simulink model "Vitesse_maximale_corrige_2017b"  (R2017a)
settings: Solver=VariableStepAuto  StartTime=0.0  StopTime=20  MinStep=0.00001  RelTol=1e-3
model workspace: external: MAT-File (data not in the file)
libraries: fl_lib x19, nesl_utility x13, sdl_lib x3, powerlib_meascontrol x3, ee_lib x3, batteryecm_lib x1

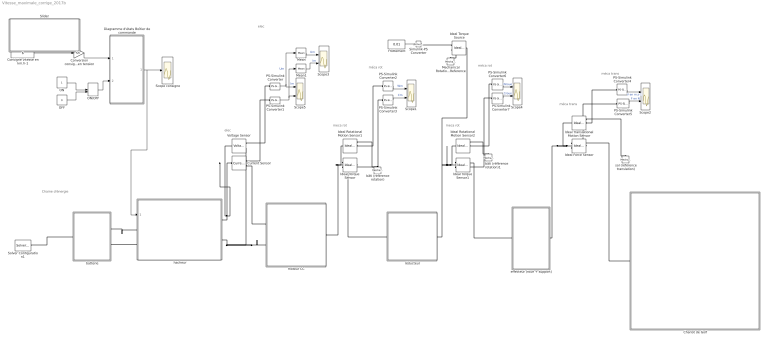
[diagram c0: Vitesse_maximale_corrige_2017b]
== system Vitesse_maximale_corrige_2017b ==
  note: méca rot
  note: méca trans
  note: meca rot
  note: elec
  note: elec
  note: meca rot
  note: Chaine d'énergie
  note: méca trans
  note: méca rot
  Chariot de Golf : Subsystem
  Consigne vitesse en km.h-1 : Constant  Value=6
  Conversion consigne en tension : Gain  Gain=5/6
  Current Sensor : fl_lib/Electrical/Electrical Sensors/Current Sensor
  Diagramme d'états Boîtier de commande : Stateflow chart  TreatAsAtomicUnit=on
  Frottement : Constant  Value=0.01
  Ideal Force Sensor : fl_lib/Mechanical/Mechanical Sensors/Ideal Force Sensor
  Ideal Rotational Motion Sensor1 : fl_lib/Mechanical/Mechanical Sensors/Ideal Rotational Motion Sensor  reference=foundation.enum.MeasurementReference.difference  acceleration_port=false  velocity_port=true  position_port=true  wrap_angle=false  offset=0 rad
  Ideal Rotational Motion Sensor2 : fl_lib/Mechanical/Mechanical Sensors/Ideal Rotational Motion Sensor  reference=foundation.enum.MeasurementReference.difference  acceleration_port=false  velocity_port=true  position_port=true  wrap_angle=false  offset=0 rad
  Ideal Torque Sensor : fl_lib/Mechanical/Mechanical Sensors/Ideal Torque Sensor
  Ideal Torque Sensor1 : fl_lib/Mechanical/Mechanical Sensors/Ideal Torque Sensor
  Ideal Torque Source : fl_lib/Mechanical/Mechanical Sources/Ideal Torque Source
  Ideal Translational Motion Sensor : fl_lib/Mechanical/Mechanical Sensors/Ideal Translational Motion Sensor  reference=foundation.enum.MeasurementReference.difference  acceleration_port=false  velocity_port=true  position_port=true  offset=0 m
  Mean : powerlib_meascontrol/Measurements/Mean  Freq=100  Vinit=24  Ts=0
  Mean1 : powerlib_meascontrol/Measurements/Mean  Freq=100  Vinit=24  Ts=0
  Mechanical Rotational Reference : fl_lib/Mechanical/Rotational Elements/Mechanical Rotational Reference
  OFF : Constant  Value=0
  ON : Constant
  ON/OFF : ManualSwitch
  PS-Simulink Converter : nesl_utility/PS-Simulink Converter  PhysicalDomain=network_engine_domain  SubClassName=ps_output  LeftPortType=input  RightPortType=output  PseudoPeriodic=off  Frequencies=[]  VectorFormat=1-D array  Unit=V  AffineConversion=off
  PS-Simulink Converter1 : nesl_utility/PS-Simulink Converter  PhysicalDomain=network_engine_domain  SubClassName=ps_output  LeftPortType=input  RightPortType=output  PseudoPeriodic=off  Frequencies=[]  VectorFormat=1-D array  Unit=A  AffineConversion=off
  PS-Simulink Converter2 : nesl_utility/PS-Simulink Converter  PhysicalDomain=network_engine_domain  SubClassName=ps_output  LeftPortType=input  RightPortType=output  PseudoPeriodic=off  Frequencies=[]  VectorFormat=1-D array  Unit=rad/s  AffineConversion=off
  PS-Simulink Converter3 : nesl_utility/PS-Simulink Converter  PhysicalDomain=network_engine_domain  SubClassName=ps_output  LeftPortType=input  RightPortType=output  PseudoPeriodic=off  Frequencies=[]  VectorFormat=1-D array  Unit=N*m  AffineConversion=off
  PS-Simulink Converter4 : nesl_utility/PS-Simulink Converter  PhysicalDomain=network_engine_domain  SubClassName=ps_output  LeftPortType=input  RightPortType=output  PseudoPeriodic=off  Frequencies=[]  VectorFormat=1-D array  Unit=m/s  AffineConversion=off
  PS-Simulink Converter5 : nesl_utility/PS-Simulink Converter  PhysicalDomain=network_engine_domain  SubClassName=ps_output  LeftPortType=input  RightPortType=output  PseudoPeriodic=off  Frequencies=[]  VectorFormat=1-D array  Unit=N  AffineConversion=off
  PS-Simulink Converter6 : nesl_utility/PS-Simulink Converter  PhysicalDomain=network_engine_domain  SubClassName=ps_output  LeftPortType=input  RightPortType=output  PseudoPeriodic=off  Frequencies=[]  VectorFormat=1-D array  Unit=rad/s  AffineConversion=off
  PS-Simulink Converter7 : nesl_utility/PS-Simulink Converter  PhysicalDomain=network_engine_domain  SubClassName=ps_output  LeftPortType=input  RightPortType=output  PseudoPeriodic=off  Frequencies=[]  VectorFormat=1-D array  Unit=N*m  AffineConversion=off
  Scope consigne : Scope
  "Scope1 " : Scope  NumInputPorts=2
  "Scope2 " : Scope  NumInputPorts=2
  "Scope3 " : Scope  NumInputPorts=2
  "Scope4 " : Scope  NumInputPorts=2
  "Scope5 " : Scope  NumInputPorts=2
  Simulink-PS Converter : nesl_utility/Simulink-PS Converter  PhysicalDomain=network_engine_domain  SubClassName=ps_input  LeftPortType=input  RightPortType=output  PseudoPeriodic=off  Frequencies=[]  NoiseDistribution=none  NoiseParameters=[]  Unit=N*m  AffineConversion=off  FilteringAndDerivatives=provide  SimscapeFilterOrder=1  InputFilterTimeConstant=0.001  UdotUserProvided=0
  Slider : Subsystem  DialogController=hmiCreateDDGDialog  IsWebBlock=on
  Solver Configuration1 : nesl_utility/Solver Configuration  PhysicalDomain=network_engine_domain  SubClassName=solver  LeftPortType=input  RightPortType=generic  Tones=[]  Harmonics=[]  SimulateNoise=off  Profile=off  UseLocalSampling=off  EnableSwitchedLinearOptims=on  FrequencyDomain=off  UseCCode=off  RelTol=0.001  AbsTol=1e-06  MinStep=1e-09  ToWorkspace=off  RevertToSquareIcSolve=off  NumHomotopyIterations=100  PhasorMode=off  PhasorModeNumHarmonics=1  ConsistencySolver=NEWTON_FTOL  IndexReductionMethod=DerivativeReplacement  DoDC=off  ResidualTolerance=1e-09  ConsistencyTolSource=GLOBAL  ConsistencyAbsTol=0.001  ConsistencyRelTol=0.001  ConsistencyTolFactor=0.001  UseLocalSolver=off  LocalSolverChoice=NE_BACKWARD_EULER_ADVANCER  ResolveIndetEquations=on  FunctionEvalNumThread=1  LocalSolverSampleTime=0.001  DoFixedCost=off  MaxNonlinIter=3  MaxModeIter=2  ComputeImpulses=off  ImpulseIterations=2  LinearAlgebra=Sparse  LinearAlgebraNumThread=0  EquationFormulation=NE_TIME_EF  DelaysMemoryBudget=1024  AutomaticFiltering=on  FilteringTimeConstant=0.001  PartitionStorageMethod=AS_NEEDED  PartitionMemoryBudget=1024  PartitionMethod=FAST  MultibodyUseLocalSolver=off  MultibodyLocalSolverChoice=ODE1  MultibodyLocalSolverSampleTime=0.001
  Voltage Sensor : fl_lib/Electrical/Electrical Sensors/Voltage Sensor
  batterie : Subsystem
  bâti (référence rotation) : fl_lib/Mechanical/Rotational Elements/Mechanical Rotational Reference
  bâti (référence rotation)1 : fl_lib/Mechanical/Rotational Elements/Mechanical Rotational Reference
  effecteur (roue + support) : Subsystem
  hacheur : Subsystem
  moteur CC : Subsystem
  réducteur : Subsystem
  sol (référence translation) : fl_lib/Mechanical/Translational Elements/Mechanical Translational Reference
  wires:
  PS-Simulink Converter1/1 -> Mean1/1, "Scope5 "/2  "Im"
  PS-Simulink Converter4/1 -> "Scope2 "/1  "V en m.s-1"
  Mean/1 -> "Scope3 "/1  "Um"
  PS-Simulink Converter/1 -> Mean/1, "Scope5 "/1  "Um"
  Mean1/1 -> "Scope3 "/2  "Im"
  PS-Simulink Converter5/1 -> "Scope2 "/2  "F en N"
  PS-Simulink Converter2/1 -> "Scope1 "/1  "Wm"
  PS-Simulink Converter6/1 -> "Scope4 "/1  "Wroue"
  PS-Simulink Converter3/1 -> "Scope1 "/2  "Cm"
  Frottement/1 -> Simulink-PS Converter/1
  PS-Simulink Converter7/1 -> "Scope4 "/2  "Croue"
  Diagramme d'états Boîtier de commande/1(consigne) -> hacheur/1(Consigne), Scope consigne/1
  ON/1 -> ON/OFF/1
  ON/OFF/1 -> Diagramme d'états Boîtier de commande/2(Bouton_marche)
  OFF/1 -> ON/OFF/2
  Conversion consigne en tension/1 -> Diagramme d'états Boîtier de commande/1(Potentiometre)
  Consigne vitesse en km.h-1/1 -> Conversion consigne en tension/1
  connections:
  hacheur/RConn2 -- moteur CC/LConn2 -- Voltage Sensor/RConn2
  Ideal Force Sensor/LConn1 -- Ideal Translational Motion Sensor/LConn1 -- effecteur (roue + support)/RConn1
  hacheur/RConn1 -- Current Sensor/LConn1 -- Voltage Sensor/LConn1
  Ideal Torque Sensor1/LConn1 -- Ideal Torque Source/LConn1 -- Ideal Rotational Motion Sensor2/LConn1 -- réducteur/RConn1
  Ideal Torque Sensor/LConn1 -- Ideal Rotational Motion Sensor1/LConn1 -- moteur CC/RConn1
  Ideal Torque Source/RConn2 -- Mechanical Rotational Reference/LConn1
  Ideal Torque Sensor1/RConn1 -- effecteur (roue + support)/LConn1
  Simulink-PS Converter/RConn1 -- Ideal Torque Source/RConn1
  Solver Configuration1/RConn1 -- batterie/LConn1
  Ideal Force Sensor/RConn2 -- PS-Simulink Converter5/LConn1
  batterie/RConn1 -- hacheur/LConn1
  Ideal Rotational Motion Sensor2/RConn1 -- bâti (référence rotation)1/LConn1
  PS-Simulink Converter7/LConn1 -- Ideal Torque Sensor1/RConn2
  Ideal Translational Motion Sensor/RConn2 -- PS-Simulink Converter4/LConn1
  Ideal Translational Motion Sensor/RConn1 -- sol (référence translation)/LConn1
  PS-Simulink Converter6/LConn1 -- Ideal Rotational Motion Sensor2/RConn2
  Current Sensor/RConn2 -- moteur CC/LConn1
  PS-Simulink Converter3/LConn1 -- Ideal Torque Sensor/RConn2
  PS-Simulink Converter2/LConn1 -- Ideal Rotational Motion Sensor1/RConn2
  Ideal Torque Sensor/RConn1 -- réducteur/LConn1
  Ideal Rotational Motion Sensor1/RConn1 -- bâti (référence rotation)/LConn1
  hacheur/LConn2 -- batterie/RConn2
  PS-Simulink Converter1/LConn1 -- Current Sensor/RConn1
  PS-Simulink Converter/LConn1 -- Voltage Sensor/RConn1
  Chariot de Golf/LConn1 -- Ideal Force Sensor/RConn1

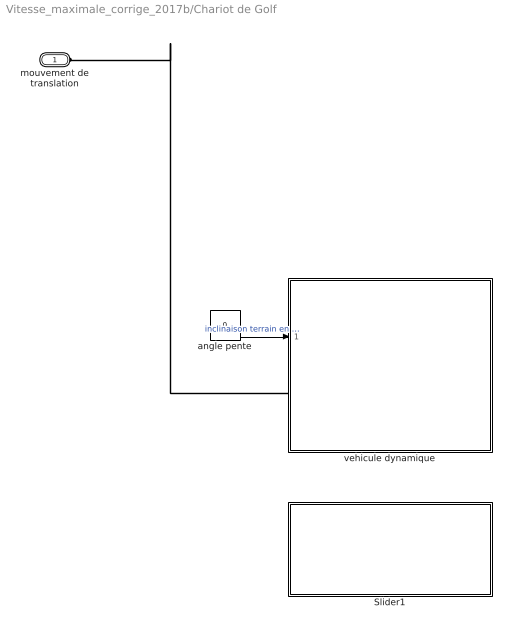
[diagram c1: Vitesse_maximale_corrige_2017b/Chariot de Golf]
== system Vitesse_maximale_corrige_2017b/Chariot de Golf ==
  Slider1 : Subsystem  DialogController=hmiCreateDDGDialog  IsWebBlock=on
  angle pente : Constant  Value=0
  vehicule dynamique : Subsystem
  mouvement de translation : PMIOPort  Side=Left
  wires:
  angle pente/1 -> vehicule dynamique/1(angle pente)  "inclinaison terrain en deg"
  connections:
  vehicule dynamique/LConn1 -- mouvement de translation/RConn1

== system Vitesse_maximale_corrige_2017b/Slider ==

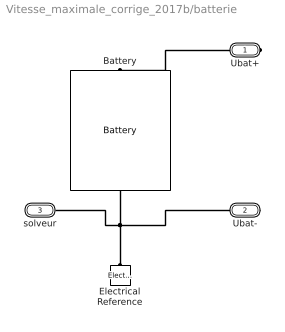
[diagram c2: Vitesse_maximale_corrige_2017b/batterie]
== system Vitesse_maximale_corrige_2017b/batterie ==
  Battery : batteryecm_lib/Battery  Vnom=16.5 V  prm_dir=simscape.enum.battery.prm_dir.disabled  R1_dis=2 Ohm  R1_ch=2 Ohm  R1=0.1 Ohm  prm_AH=2  AH=16 hr*A  V1=11.84 V  AH1=12.8 hr*A  prm_R2=2  R2=inf Ohm  Tmeas=298.15 K  charge_measurement_port=simscape.enum.battery.enable.no  prm_dyn=1  Rp1=0.005 Ohm  tau1=30 s  Rp2=0.005 Ohm  tau2=30 s  Rp3=0.005 Ohm  tau3=30 s  Rp4=0.005 Ohm  tau4=30 s  Rp5=0.005 Ohm  tau5=30 s  prm_fade=1  N_fade=100  AH_fade=45 hr*A  R1_fade=2.02 Ohm  R1_ch_fade=2.02 Ohm  V1_fade=10.35 V  prm_age=simscape.enum.battery.prm_age.disabled  prm_age_OCV=simscape.enum.battery.prm_age_OCV.OCV  OCV_age=0.9  SOC_age=60  Tmeas_age=298.15 K  delta_time_age_vec=[0] d  temperature_age_vec=[273] K  OCV_scaling_age=2.2134e6  OCV_offset_age=1.632e6  temp_exp_age=0.515833569 V  t_exp_age=0.75  Vnom_T2=12 V  R1_T2=2.2 Ohm  R1_T2_dis=2.2 Ohm  R1_T2_ch=2.2 Ohm  V1_T2=11.4 V  R2_T2=2200 Ohm  Rp1_T2=0.005 Ohm  tau1_T2=30 s  Rp2_T2=0.005 Ohm  tau2_T2=30 s  Rp3_T2=0.005 Ohm  tau3_T2=30 s  Rp4_T2=0.005 Ohm  tau4_T2=30 s  Rp5_T2=0.005 Ohm  tau5_T2=30 s  Tmeas2=273.15 K  thermal_port=simscape.enum.thermaleffects.omit  thermal_mass=30000 J/K  i_specify=off  i_priority=None  i=0 A  i_nominal_specify=off  i_nominal_unit=A  i_nominal_value=1  v_specify=off  v_priority=None  v=0 V  v_nominal_specify=off  v_nominal_unit=V  v_nominal_value=1  charge_specify=on  charge_priority=High  charge=17 hr*A  charge_nominal_specify=off  charge_nominal_unit=A*hr  charge_nominal_value=1  num_cycles_specify=on  num_cycles_priority=High  num_cycles=1  num_cycles_nominal_specify=off  num_cycles_nominal_unit=1  num_cycles_nominal_value=1  temperature_specify=off  temperature_priority=High  temperature=298.15 K  temperature_nominal_specify=off  temperature_nominal_unit=K  temperature_nominal_value=1
  Electrical Reference : fl_lib/Electrical/Electrical Elements/Electrical Reference
  Ubat+ : PMIOPort  Side=Right
  Ubat- : PMIOPort  Port=2  Side=Right
  solveur : PMIOPort  Port=3  Side=Left
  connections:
  Electrical Reference/LConn1 -- solveur/RConn1 -- Ubat-/RConn1 -- Battery/RConn1
  Ubat+/RConn1 -- Battery/LConn1

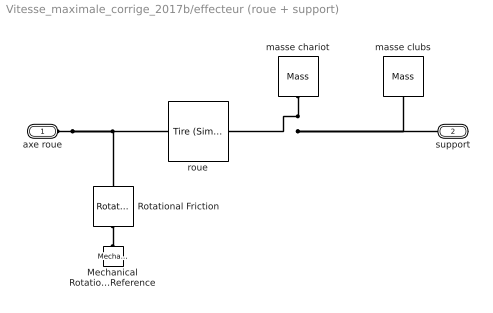
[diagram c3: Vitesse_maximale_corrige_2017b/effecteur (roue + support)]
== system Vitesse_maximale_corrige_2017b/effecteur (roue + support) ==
  Mechanical Rotational Reference : fl_lib/Mechanical/Rotational Elements/Mechanical Rotational Reference
  "Rotational Friction " : fl_lib/Mechanical/Rotational Elements/Rotational Friction  brkwy_trq=0.1 N*m  brkwy_vel=0.1 rad/s  Col_trq=0.1 N*m  visc_coef=0.0001 N*m/(rad/s)  w_specify=off  w_priority=None  w=0 rad/s  w_nominal_specify=off  w_nominal_unit=rad/s  w_nominal_value=1  t_specify=off  t_priority=None  t=0 N*m  t_nominal_specify=off  t_nominal_unit=N*m  t_nominal_value=1
  masse clubs : fl_lib/Mechanical/Translational Elements/Mass  mass=4 kg  num_ports=foundation.enum.numPorts2.one  v_specify=off  v_priority=High  v=0 m/s  v_nominal_specify=off  v_nominal_unit=m/s  v_nominal_value=1  f_specify=off  f_priority=High  f=0 N  f_nominal_specify=off  f_nominal_unit=N  f_nominal_value=1
  masse chariot : fl_lib/Mechanical/Translational Elements/Mass  mass=13.5 kg  num_ports=foundation.enum.numPorts2.one  v_specify=off  v_priority=High  v=0 m/s  v_nominal_specify=off  v_nominal_unit=m/s  v_nominal_value=1  f_specify=off  f_priority=High  f=0 N  f_nominal_specify=off  f_nominal_unit=N  f_nominal_value=1
  roue : sdl_lib/Tires & Vehicles/Tire (Simple)  r_tire=27/2 cm  model_compliance=0  stiffness=1e+6 N/m  damping=1000 N/(m/s)  model_inertia=0  tire_inertia=1 kg*m^2  initial_velocity=0 rad/s
  axe roue : PMIOPort  Side=Left
  support : PMIOPort  Port=2  Side=Right
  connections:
  masse chariot/LConn1 -- support/RConn1 -- masse clubs/LConn1 -- roue/RConn1
  axe roue/RConn1 -- roue/LConn1 -- "Rotational Friction "/LConn1
  "Rotational Friction "/RConn1 -- Mechanical Rotational Reference/LConn1

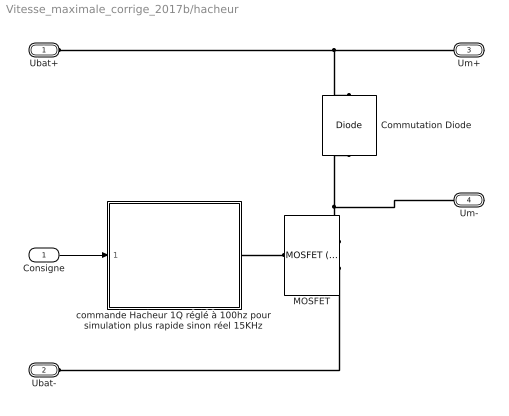
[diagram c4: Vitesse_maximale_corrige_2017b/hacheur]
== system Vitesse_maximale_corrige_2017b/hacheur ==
  Consigne : Inport
  Commutation Diode : ee_lib/Semiconductors & Converters/Diode  ModelType=ee.enum.diode.modelType.pwl  TableType=ee.enum.diode.tableType.IfMat  IfMat=[.07, .12, .19, 1.75, 4.24, 7.32, 11.2; .16, .3, .72, 2.14, 5.02, 8.35, 13.12] A  VfMat=[.9, 1.15, 1.25, 1.5, 1.75, 2.17, 2.6, 2.85; .58, .68, .75, 1.1, 1.38, 1.77, 2.27, 2.7] V  TjVec=[25, 125] degC  VfVec=[.5, .7, .9, 1.3, 1.7, 2.1, 2.5] V  IfVec=[.1, .2, .5, 1, 2, 4, 7, 10] A  Vf=0.8 V  Ron=0.001 Ohm  Goff=1e-5 1/Ohm  prmExp=ee.enum.diode.expParam.useTwo  I12=[.0137, .545] A  V12=[.6, .7] V  RS=0 Ohm  Tmeas=25 degC  IS=1e-12 A  ec=1  I1=0.0137 A  V1=0.6 V  N_series=1  N_parallel=1  ZenerEnable=false  Rz=0.3 Ohm  BV=inf V  C_param=ee.enum.diode.capParam.fixed  CJ=50 pF  CJ0=5 pF  Vvec=[.1, 10, 100] V  Cvec=[3.5, 1, .4] pF  VJ=1 V  Mgrad=0.5  FC=0.5  Q_param=1  iRM=-235 A  iF=300 A  didt=-50 A/us  trr_factor=3  trr=15 us  Qrr=1.5e+3 s*uA  Vr=-600 V  Ls=150 nH  Erec=0.03 J  TT=50 ns  tau=100 ns  T_param=ee.enum.diode.temperatureParam.off  Tdevice=25 degC  I1_T2=0.245 A  V1_T2=0.5 V  IS_T2=1.25e-7 A  Tmeas2=125 degC  XTI_param=ee.enum.diode.xtiParam.pn  XTI=3  EG_param=ee.enum.diode.egapParam.material_si  EG=1.11 eV  dBVdT=0 V/K  enable_faults=ee.enum.enable.no  fault_action=simscape.enum.assert.action.none  fault_types=ee.enum.diode.faults.open  tau_fault=1e-3 s  IfMat_faulted=[.07, .12, .19, 1.75, 4.24, 7.32, 11.2; .16, .3, .72, 2.14, 4.02, 6.35, 9.12] A  VfMat_faulted=[.9, 1.15, 1.25, 1.5, 1.75, 2.17, 2.6, 2.85; .58, .68, .75, 1.1, 1.38, 1.77, 2.27, 2.7] V  VfVec_faulted=[.5, .7, .9, 1.3, 1.7, 2.1, 2.5] V  IfVec_faulted=[.1, .2, .5, 1, 2, 4, 7, 10] A  Ropen_faulted=1000 Ohm  Gshort_faulted=1000 1/Ohm  Vf_faulted=0.6 V  Ron_faulted=0.3 Ohm  Goff_faulted=1e-8 S  I12_faulted=[.0137, .545] A  V12_faulted=[.6, .7] V  IS_faulted=1e-12 A  ec_faulted=1  I1_faulted=0.0137 A  V1_faulted=0.6 V  RS_faulted=0 Ohm  Rz_faulted=0.3 Ohm  BV_faulted=inf V  Cscale_faulted=100  fault_trigger=ee.enum.faults.faultTrigger.temporal  t_fault=inf s  max_permissible_voltage=inf V  n_fail_on_voltage=1  max_permissible_current=inf A  t_fail_on_current=1 s  max_permissible_dVdt=inf V/s  enable_fault_input=simscape.enum.onoff.off  i_specify=off  i_priority=None  i=0 A  i_nominal_specify=off  i_nominal_unit=A  i_nominal_value=1  v_specify=off  v_priority=None  v=0 V  v_nominal_specify=off  v_nominal_unit=V  v_nominal_value=1  v_capacitor_specify=off  v_capacitor_priority=None  v_capacitor=0 V  v_capacitor_nominal_specify=off  v_capacitor_nominal_unit=V  v_capacitor_nominal_value=1  faulted_specify=off  faulted_priority=None  faulted=0  faulted_nominal_specify=off  faulted_nominal_unit=1  faulted_nominal_value=1  i_diode_specify=off  i_diode_priority=None  i_diode=0 A  i_diode_nominal_specify=off  i_diode_nominal_unit=A  i_diode_nominal_value=1  v_diode_specify=off  v_diode_priority=None  v_diode=0 V  v_diode_nominal_specify=off  v_diode_nominal_unit=V  v_diode_nominal_value=1  i_capacitor_specify=off  i_capacitor_priority=None  i_capacitor=0 A  i_capacitor_nominal_specify=off  i_capacitor_nominal_unit=A  i_capacitor_nominal_value=1  power_dissipated_specify=off  power_dissipated_priority=None  power_dissipated=0 W  power_dissipated_nominal_specify=off  power_dissipated_nominal_unit=W  power_dissipated_nominal_value=1  fidelity_level=ee.enum.diode.fidelity.includeChargeDyn  rec_loss_model=ee.enum.diode.reverseRecoveryModel.fixed  ErecVal=0 J  scaleWithIandV=true  ErecMat=zeros(2, 3) J  TjrecVec=[298.15, 398.15] K  IfrecVec=[.1, 1, 10] A  IrecVal=10 A  VrecVal=10 V  tFilter=1 / 1000 / 100 s  max_permissible_temperature=inf K  t_fail_on_temperature=1 s  thermal_network_parameterization=ee.enum.thermalNetworkTopology.junctionCase  Rth=[0, 10] K/W  Rth_Cauer=[1, 3, 10] K/W  Rth_Foster=[4, 6] K/W  thermal_mass_parameterization=ee.enum.thermalNetwork.timeconstant  thermal_mass=[0, 1] J/K  thermal_mass_Cauer=[.1, .3, 1] J/K  thermal_mass_Foster=[1.5, 3] J/K  thermal_time_constant=[0, 10] s  thermal_time_constant_Cauer=[1, 3, 10] s  thermal_time_constant_Foster=[6, 18] s  thermal_mass_initial_temperatures=[25, 25] degC  thermal_mass_initial_temperatures_Cauer=[25, 25, 25] degC  junction_thermal_mass=0.01 J/K  Tvec_initial_Foster=[25, 25, 25, 25] degC  no_thermal_network=0  junction_temperature_specify=off  junction_temperature_priority=None  junction_temperature=25 degC  junction_temperature_nominal_specify=off  junction_temperature_nominal_unit=degC  junction_temperature_nominal_value=1
  MOSFET : ee_lib/Semiconductors & Converters/MOSFET (Ideal, Switching)  port_option=ee.enum.controlport.ps  Rds=0.01 Ohm  Goff=1e-6 1/Ohm  Vth=2 V  diode_param=2  diode_Vf=0.8 V  diode_Ron=0.001 Ohm  diode_Goff=1e-5 1/Ohm  diode_C=5e-8 F  diode_iRM=-235 A  diode_iF=300 A  diode_idot=-50 A/us  diode_trr_param=1  diode_trr_factor=3  diode_trr=15 us  diode_Qrr=1.5e+3 s*uA  ids_specify=off  ids_priority=None  ids=0 A  ids_nominal_specify=off  ids_nominal_unit=A  ids_nominal_value=1  vds_specify=off  vds_priority=None  vds=0 V  vds_nominal_specify=off  vds_nominal_unit=V  vds_nominal_value=1  vgs_specify=off  vgs_priority=None  vgs=0 V  vgs_nominal_specify=off  vgs_nominal_unit=V  vgs_nominal_value=1  thermal_loss_option=ee.enum.converters.thermalLossOption.constantvalues  Von_data=[0, 1.8, 3.2, 6, 10, 16; 0, 2, 5.5, 9.5, 15, 25] V  Tj=[298.15, 448.15] K  Iout_data=[0, 20, 40, 60, 80, 100] A  Eon_data=[0, 55.04, 124.57, 235.53, 362.12; 0, 71.25, 161.25, 304.88, 468.75] * 1e-6 J  Eoff_data=[0, 18, 30, 56.1, 76.5; 0, 22.5, 37.5, 70.13, 95.63] * 1e-6 J  Eon_data_3D=[zeros(2, 5, 3)] J  Eoff_data_3D=[zeros(2, 5, 3)] J  Tj_loss=[298.15, 448.15] K  Iout_data_loss=[0, 10, 20, 30, 40] A  tabulateWithVds=false  Vds_loss=[0, 150, 300] V  Eon_scalar=22.86e-3 J  Eoff_scalar=17.14e-3 J  Voff=300 V  Iout_scalar=600 A  useCurrentFromPreviousCycle=false  useVoltageFromPreviousCycle=false  diodeModelType=ee.enum.converters.diodeModelType.pwl  diodeTableType=ee.enum.diode.tableType.IfMat  diode_IfMat=[.07, .12, .19, 1.75, 4.24, 7.32, 11.2; .16, .3, .72, 2.14, 4.02, 6.35, 9.12] A  diode_VfMat=[.9, 1.15, 1.25, 1.5, 1.75, 2.17, 2.6, 2.85; .58, .68, .75, 1.1, 1.38, 1.77, 2.27, 2.7] V  diode_TjVec=[25, 125] degC  diode_VfVec=[.5, .7, .9, 1.3, 1.7, 2.1, 2.5] V  diode_IfVec=[.1, .2, .5, 1, 2, 4, 7, 10] A  diode_Vr=-600 V  diode_Ls=150 nH  diode_Erec=0.03 J  diode_rec_loss_model=ee.enum.diode.reverseRecoveryModel.fixed  diode_ErecVal=0 J  diode_scaleWithIandV=true  diode_ErecMat=zeros(2, 3) J  diode_TjrecVec=[298.15, 398.15] K  diode_IfrecVec=[.1, 1, 10] A  diode_IrecVal=10 A  diode_VrecVal=10 V  diode_tFilter=1 / 1000 / 100 s  thermal_network_parameterization=ee.enum.thermalNetworkTopology.external  Rth=[.03, .2] K/W  Rth_Cauer=[.03, .1, .2] K/W  Rth_Foster=[.03, .2] K/W  thermal_mass_parameterization=ee.enum.thermalNetwork.timeconstant  thermal_mass=[3, 25] J/K  thermal_mass_Cauer=[3, 10, 25] J/K  thermal_mass_Foster=[33, 50] J/K  thermal_time_constant=[.1, 5] s  thermal_time_constant_Cauer=[.1, 1, 5] s  thermal_time_constant_Foster=[1, 10] s  thermal_mass_initial_temperatures=[25, 25] degC  thermal_mass_initial_temperatures_Cauer=[25, 25, 25] degC  junction_thermal_mass=0.1 J/K  Tvec_initial_Foster=[25, 25, 25, 25] degC  no_thermal_network=0  junction_temperature_specify=off  junction_temperature_priority=None  junction_temperature=25 degC  junction_temperature_nominal_specify=off  junction_temperature_nominal_unit=degC  junction_temperature_nominal_value=1  Qj_specify=off  Qj_priority=None  Qj=0 W  Qj_nominal_specify=off  Qj_nominal_unit=W  Qj_nominal_value=1  accumulatedSwitchingLosses_specify=off  accumulatedSwitchingLosses_priority=None  accumulatedSwitchingLosses=0 J
  commande Hacheur 1Q réglé à 100hz pour simulation plus rapide sinon réel 15KHz : Subsystem
  Ubat+ : PMIOPort  Side=Left
  Ubat- : PMIOPort  Port=2  Side=Left
  Um+ : PMIOPort  Port=3  Side=Right
  Um- : PMIOPort  Port=4  Side=Right
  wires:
  Consigne/1 -> commande Hacheur 1Q réglé à 100hz pour simulation plus rapide sinon réel 15KHz/1(consigne)
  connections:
  Ubat+/RConn1 -- Um+/RConn1 -- Commutation Diode/RConn1
  MOSFET/RConn1 -- Commutation Diode/LConn1 -- Um-/RConn1
  MOSFET/LConn1 -- commande Hacheur 1Q réglé à 100hz pour simulation plus rapide sinon réel 15KHz/RConn1
  MOSFET/RConn2 -- Ubat-/RConn1

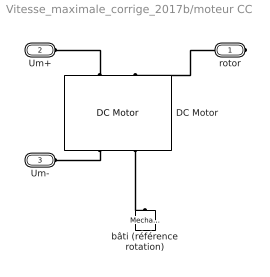
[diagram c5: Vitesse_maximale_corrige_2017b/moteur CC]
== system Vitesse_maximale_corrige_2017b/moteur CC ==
  DC Motor : ee_lib/Electromechanical/Brushed Motors/DC Motor  field_option=ee.enum.field_option.pm  Rf=100 Ohm  Lf=1 H  Laf=0.15 H  If0=0 A  parameterization=1  Ra=0.54 Ohm  La=12e-3 H  emf_or_torque=1  Kv=2.9e-3 V/rpm  Ki=6.876e-4 N*m/A  T_stall=2.4e-4 N*m  w_max=3800 rpm  w_rated=3800 rpm  P_rated=150 W  V_rated=12 V  lam_param=1  i_noload=1 A  V_i_noload=12 V  J=0.0001 kg*m^2  lam=0.0001 N*m/(rad/s)  speed0=0 rpm  enable_fault_armature=simscape.enum.onoff.off  rev_faulted=1 / 3  G_faulted_armature=1e-5 S  fault_trigger_armature=ee.enum.faults.faultTrigger.temporal  t_fault_armature=1 s  max_permissible_current_armature=inf A  t_fail_on_current_armature=1 s  enable_fault_field=simscape.enum.onoff.off  G_faulted_field=1e-5 S  fault_trigger_field=ee.enum.faults.faultTrigger.temporal  t_fault_field=1 s  max_permissible_current_field=inf A  t_fail_on_current_field=1 s  fault_action=simscape.enum.assert.action.none  alpha=3.93e-3 1/K  Tmeas=25 degC  thermal_mass=100 J/K  initial_temperature=25 degC
  bâti (référence rotation) : fl_lib/Mechanical/Rotational Elements/Mechanical Rotational Reference
  rotor : PMIOPort  Side=Right
  Um+ : PMIOPort  Port=2  Side=Left
  Um- : PMIOPort  Port=3  Side=Left
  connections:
  rotor/RConn1 -- DC Motor/LConn2
  DC Motor/RConn2 -- bâti (référence rotation)/LConn1
  DC Motor/RConn1 -- Um-/RConn1
  DC Motor/LConn1 -- Um+/RConn1

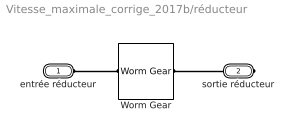
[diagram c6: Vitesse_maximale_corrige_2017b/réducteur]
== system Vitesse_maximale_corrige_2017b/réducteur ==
  Worm Gear : sdl_lib/Gears/Worm Gear  ratio=25/1  thread_type=1  friction_model=2  friction_parameterization=1  pr_ang=20 deg  lead_ang=74.534 deg  fr_coeff=0.08  eff_wg=0.74  eff_gw=0.65  temperature_TLU=[280, 300, 320] K  efficiency_wg_TLU=[.75, .65, .6]  efficiency_gw_TLU=[.5, .45, .4]  pwr_thr=0.001 W  mu_visc=[0, 0] N*m/(rad/s)  thermal_mass=50 J/K  temperature_specify=off  temperature_priority=High  temperature=300 K  temperature_nominal_specify=off  temperature_nominal_unit=K  temperature_nominal_value=1
  entrée réducteur : PMIOPort  Side=Left
  sortie réducteur : PMIOPort  Port=2  Side=Right
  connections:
  entrée réducteur/RConn1 -- Worm Gear/LConn1
  Worm Gear/RConn1 -- sortie réducteur/RConn1

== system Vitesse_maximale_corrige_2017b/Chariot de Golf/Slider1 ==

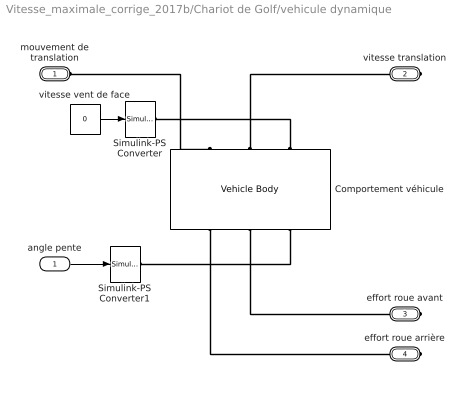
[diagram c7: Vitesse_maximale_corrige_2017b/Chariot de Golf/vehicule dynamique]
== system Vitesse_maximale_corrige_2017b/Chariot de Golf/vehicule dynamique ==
  angle pente : Inport  OutMin=[0]  OutMax=[20000]
  Comportement véhicule : sdl_lib/Tires & Vehicles/Vehicle Body  mass=17.5 kg  n_w=1  x_f=580 mm  x_r=60 mm  y_c=24+27/2 cm  mass_var=simscape.enum.onoff.off  g=9.81 m/s^2  liftoff_warning=0  area=0.52828 m^2  Cd=1  rho=1.24 kg/m^3  model_pitch=0  inertia=4000 kg*m^2  suspension_model=1  k_f=1e4 N/m  b_f=1e4 N/(m/s)  k_r=1e4 N/m  b_r=1e4 N/(m/s)  k_f_TLU=[-2000, -1000, 0, 1000, 2000] N  x_f_TLU=[-.4, -.2, 0, .2, .4] m  b_f_TLU=[-200, -100, 0, 100, 200] N  v_f_TLU=[-4, -2, 0, 2, 4] m/s  k_r_TLU=[-2000, -1000, 0, 1000, 2000] N  x_r_TLU=[-.4, -.2, 0, .2, .4] m  b_r_TLU=[-200, -100, 0, 100, 200] N  v_r_TLU=[-4, -2, 0, 2, 4] m/s  interp_method=simscape.enum.interpolation.linear  extrap_method=simscape.enum.extrapolation.linear  model_hardstop=0  upper_bound_f=.25 m  lower_bound_f=-.25 m  stop_k_f=1e6 N/m  stop_b_f=150 N/(m/s)  upper_bound_r=.25 m  lower_bound_r=-.25 m  stop_k_r=1e6 N/m  stop_b_r=150 N/(m/s)  initial_pitch=0 rad  initial_pitch_rate=0 rad/s  v_specify=on  v_priority=High  v=0 m/s  v_nominal_specify=off  v_nominal_unit=m/s  v_nominal_value=1
  Simulink-PS Converter : nesl_utility/Simulink-PS Converter  PhysicalDomain=network_engine_domain  SubClassName=ps_input  LeftPortType=input  RightPortType=output  PseudoPeriodic=off  Frequencies=[]  NoiseDistribution=none  NoiseParameters=[]  Unit=m/s  AffineConversion=off  FilteringAndDerivatives=zero  SimscapeFilterOrder=1  InputFilterTimeConstant=0.001  UdotUserProvided=1
  Simulink-PS Converter1 : nesl_utility/Simulink-PS Converter  PhysicalDomain=network_engine_domain  SubClassName=ps_input  LeftPortType=input  RightPortType=output  PseudoPeriodic=off  Frequencies=[]  NoiseDistribution=none  NoiseParameters=[]  Unit=deg  AffineConversion=off  FilteringAndDerivatives=zero  SimscapeFilterOrder=1  InputFilterTimeConstant=0.001  UdotUserProvided=1
  vitesse vent de face : Constant  Value=0
  mouvement de translation : PMIOPort  Side=Left
  vitesse translation : PMIOPort  Port=2  Side=Right
  effort roue avant : PMIOPort  Port=3  Side=Right
  effort roue arrière : PMIOPort  Port=4  Side=Right
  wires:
  vitesse vent de face/1 -> Simulink-PS Converter/1
  angle pente/1 -> Simulink-PS Converter1/1
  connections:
  mouvement de translation/RConn1 -- Comportement véhicule/LConn1
  Simulink-PS Converter/RConn1 -- Comportement véhicule/LConn3
  Comportement véhicule/LConn2 -- vitesse translation/RConn1
  Comportement véhicule/RConn2 -- effort roue avant/RConn1
  Comportement véhicule/RConn1 -- effort roue arrière/RConn1
  Simulink-PS Converter1/RConn1 -- Comportement véhicule/RConn3

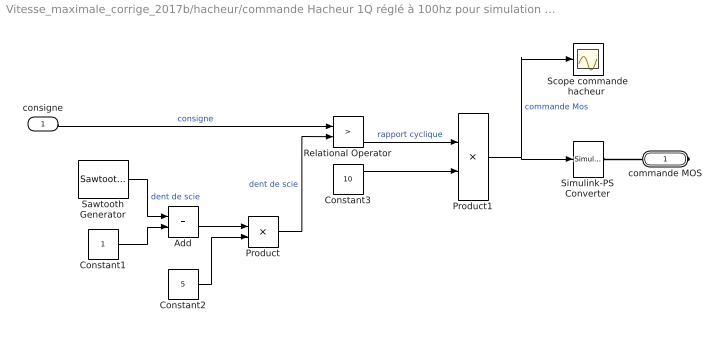
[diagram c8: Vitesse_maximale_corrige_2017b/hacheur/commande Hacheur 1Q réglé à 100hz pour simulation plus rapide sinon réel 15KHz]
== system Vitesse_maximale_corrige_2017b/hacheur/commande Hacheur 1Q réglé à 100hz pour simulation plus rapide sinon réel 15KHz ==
  consigne : Inport
  Add : Sum
  Constant1 : Constant  OutMin=[0]  OutMax=[10]
  Constant2 : Constant  Value=5  OutMin=[0]  OutMax=[10]
  Constant3 : Constant  Value=10  OutMin=[0]  OutMax=[10]
  Product : Product
  Product1 : Product  OutDataTypeStr=double
  Relational Operator : RelationalOperator  Operator=>  OutDataTypeStr=boolean
  Sawtooth Generator : powerlib_meascontrol/Pulse & Signal Generators/Sawtooth Generator  Freq=100  Phase=0  Ts=0
  "Scope commande hacheur " : Scope
  Simulink-PS Converter : nesl_utility/Simulink-PS Converter  PhysicalDomain=network_engine_domain  SubClassName=ps_input  LeftPortType=input  RightPortType=output  PseudoPeriodic=off  Frequencies=[]  NoiseDistribution=none  NoiseParameters=[]  Unit=V  AffineConversion=off  FilteringAndDerivatives=zero  SimscapeFilterOrder=1  InputFilterTimeConstant=0.001  UdotUserProvided=1
  commande MOS : PMIOPort  Side=Right
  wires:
  Product/1 -> Relational Operator/2  "dent de scie"
  Constant2/1 -> Product/2
  Sawtooth Generator/1 -> Add/1  "dent de scie"
  Constant1/1 -> Add/2
  Add/1 -> Product/1
  Relational Operator/1 -> Product1/1  "rapport cyclique"
  Constant3/1 -> Product1/2
  Product1/1 -> "Scope commande hacheur "/1, Simulink-PS Converter/1  "commande Mos"
  consigne/1 -> Relational Operator/1  "consigne"
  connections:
  Simulink-PS Converter/RConn1 -- commande MOS/RConn1

== stateflow chart Vitesse_maximale_corrige_2017b/Diagramme d'états 
Boîtier de commande ==
  state Marche
    entry: consigne=Potentiometre;
  state arret
    en, du: consigne=0;
  (default) -> arret
  Marche -> arret : [Bouton_marche==0]
  arret -> Marche : [Bouton_marche==1]
  data: consigne output; i local; temps local; Potentiometre input; Bouton_marche input
